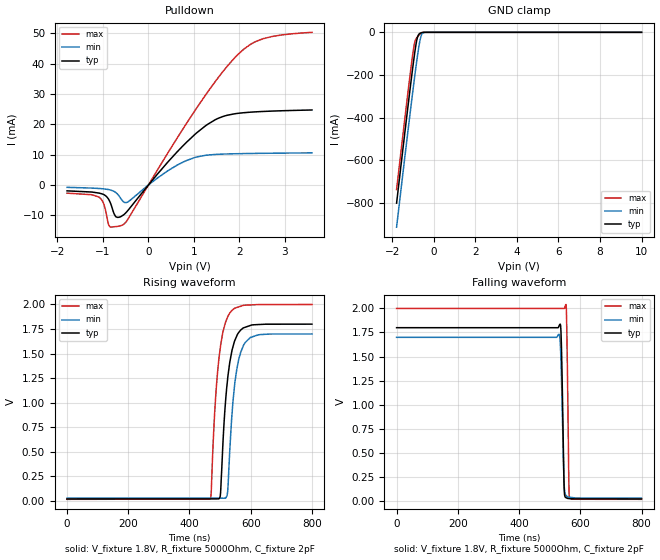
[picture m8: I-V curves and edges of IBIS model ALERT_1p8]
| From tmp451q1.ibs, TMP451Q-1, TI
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|   Model
[Model]   ALERT_1p8
Model_type   Open_drain
Polarity   Non-Inverting
Vmeas = 0.9
Vref = 1.8
Cref = 2pF
Rref = 5000
|   typ   min   max
C_comp   1.79pF   1.73pF   1.91pF
[Voltage Range]   1.8   1.7   2
[Temperature Range]   25   125   -40
[Pullup Reference]   1.8   1.7   2
[Pulldown Reference]   0   0   0
[Power Clamp Reference]   1.8   1.7   2
[GND Clamp Reference]   0   0   0
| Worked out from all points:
|   slope of the pulldown table from 0 to 0.27 V, typ, clamps not added: 55.8 ohm
|   GND clamp passes 1 mA (typ) near -0.56 V on its own axis
|   falling waveform, V_fixture 1.8V, R_fixture 5000Ohm, C_fixture 2pF: 20-80 % time 6.08ns typ, 7.64ns min, 4.94ns max; typ from 1.8 V to 0.019 V
|   rising waveform, V_fixture 1.8V, R_fixture 5000Ohm, C_fixture 2pF: 20-80 % time 27.4ns typ, 27ns min, 27.7ns max; typ from 0.019 V to 1.8 V
[Pulldown]
|   Voltage   I(typ)   I(min)   I(max)
-1.79V    -1.932mA   -771.8uA   -2.683mA
-1.085V   -2.673mA   -1.148mA   -3.986mA
-980mV    -3.169mA   -1.287mA   -6.323mA
-845mV    -5.581mA   -1.61mA    -13.82mA
-725mV    -10.3mA    -2.395mA   -13.71mA
-545mV    -9.832mA   -5.592mA   -12.95mA
445mV     7.859mA    4.862mA    10.99mA
1.015V    16.56mA    9.027mA    24.34mA
1.465V    21.46mA    10.05mA    33.99mA
1.93V     23.52mA    10.3mA     42.41mA
2.515V    24.21mA    10.43mA    48.14mA
3.595V    24.7mA     10.58mA    50.28mA
[GND Clamp]
|   Voltage   I(typ)   I(min)   I(max)
-1.79V    -800.3mA   -912.7mA   -736.5mA
-1.235V   -341.3mA   -456.3mA   -275.1mA
-1.07V    -210.1mA   -324.5mA   -145.2mA
-965mV    -130.5mA   -242.7mA   -72.22mA
-890mV    -78.25mA   -185.9mA   -38.18mA
-830mV    -42.99mA   -142mA     -27.13mA
-770mV    -19.04mA   -100.5mA   -19.54mA
-695mV    -7.009mA   -54.42mA   -11.27mA
-635mV    -3.322mA   -25.87mA   -6.076mA
-590mV    -1.668mA   -11.94mA   -3.161mA
-530mV    -477.6uA   -3.298mA   -844.4uA
10V       0A         0A         0A
[Ramp]
R_load = 5000
|   typ   min   max
dV/dt_r   1.06838/2.71832e-08   1.00325/2.67966e-08   1.19052/2.76905e-08
dV/dt_f   1.06838/6.07586e-09   1.00325/7.6427e-09   1.19052/4.93512e-09
[Falling Waveform]
V_fixture = 1.8V
V_fixture_min = 1.7V
V_fixture_max = 2V
R_fixture = 5000Ohm
C_fixture = 2pF
|   Time   V(typ)   V(min)   V(max)
0s        1.8V       1.7V       2V
531ns     1.82V      1.732V     2V
534.8ns   1.836V     1.625V     2V
538.7ns   1.57V      1.249V     2V
547.4ns   131.1mV    167.2mV    2V
553.2ns   33.04mV    55.64mV    2.041V
556.2ns   28.8mV     46.56mV    1.724V
562.9ns   24.08mV    38.08mV    146mV
565ns     23.6mV     37.32mV    30.54mV
800ns     19.37mV    27.91mV    15.8mV
[Rising Waveform]
V_fixture = 1.8V
V_fixture_min = 1.7V
V_fixture_max = 2V
R_fixture = 5000Ohm
C_fixture = 2pF
|   Time   V(typ)   V(min)   V(max)
0s        19.37mV    27.91mV    15.8mV
467ns     20.43mV    27.37mV    18.62mV
471ns     20.44mV    27.36mV    88.19mV
486.6ns   20.48mV    27.35mV    1.109V
500.3ns   46.99mV    27.33mV    1.551V
513.9ns   843.8mV    27.31mV    1.775V
525.6ns   1.271V     133.1mV    1.88V
547.7ns   1.631V     1.188V     1.962V
576.5ns   1.762V     1.584V     1.992V
800ns     1.8V       1.7V       2V
